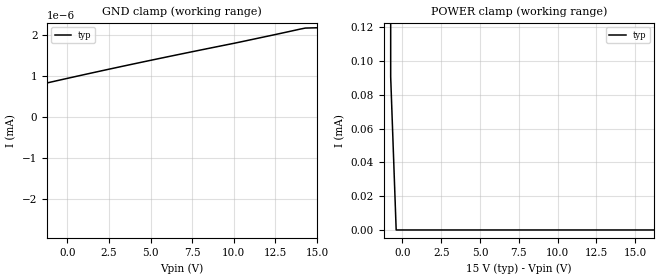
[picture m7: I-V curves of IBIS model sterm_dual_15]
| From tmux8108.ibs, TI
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| sterm_dual_15
[Model]   sterm_dual_15
Model_type   Terminator
|   typ   min   max
C_comp   4.014581e-12   NA   NA
[Voltage Range]   15   NA   NA
[Temperature Range]   27   NA   NA
[Power Clamp Reference]   15   NA   NA
[GND Clamp Reference]   0   NA   NA
[GND Clamp]
|   Voltage   I(typ)   I(min)   I(max)
-20V      -1.144A    NA         NA
-15.4V    -86.76nA   NA         NA
-15.05V   -296.1pA   NA         NA
-12.22V   -129.7pA   NA         NA
-9.747V   51.91pA    NA         NA
4.394V    1.328nA    NA         NA
14.29V    2.163nA    NA         NA
15V       2.17nA     NA         NA
[POWER Clamp]
|   Voltage   I(typ)   I(min)   I(max)
-5V       744mA      NA         NA
-1.111V   26.13mA    NA         NA
-757.6mV  90.5uA     NA         NA
-404mV    2.534nA    NA         NA
30V       -293pA     NA         NA
